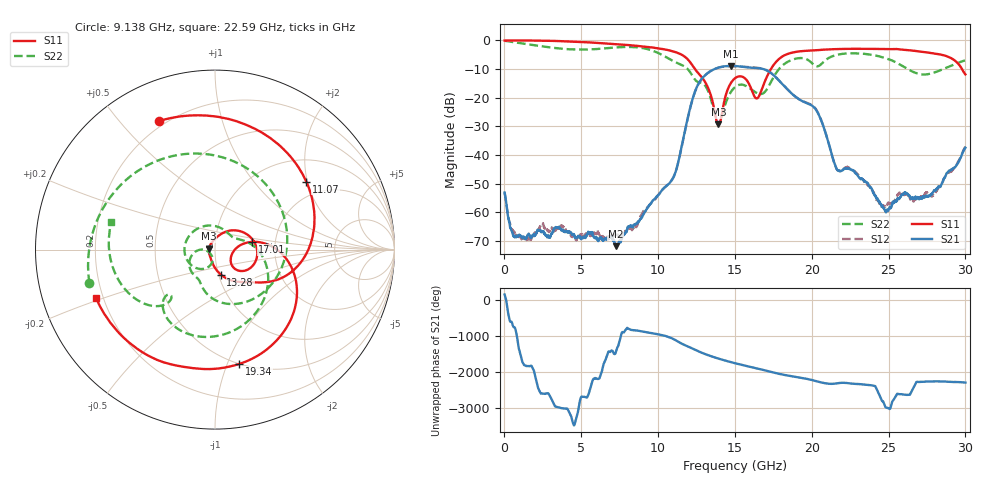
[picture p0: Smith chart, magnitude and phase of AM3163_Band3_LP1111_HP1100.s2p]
!Agilent Technologies,E8364B,MY43040894,A.07.50.67
!Agilent E8364B: A.07.50.67
!Date: Thursday, August 20, 2020 12:17:28
!Correction: S11(Full 2 Port(1,2))
!S21(Full 2 Port(1,2))
!S12(Full 2 Port(1,2))
!S22(Full 2 Port(1,2))
!S2P File: Measurements: S11, S21, S12, S22:
# Hz S  dB  R 50
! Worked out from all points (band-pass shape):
!   3201 points, 10 MHz to 30 GHz, reference 50 ohm
!   highest |S21| = -8.87 dB at 14.75 GHz (marker M1); lowest = -71.7 dB at 7.245 GHz (marker M2)
!   |S21| within 3 dB of the highest: 13.12 GHz to 17.47 GHz (4.35 GHz wide, 28.4 % of centre)
!   lowest |S11| = -29.3 dB at 13.93 GHz (marker M3), VSWR 1.07, Z = 46.7 + j0.464 ohm
!   |S11| at or under -10 dB: 12.41 GHz to 17.34 GHz (4.934 GHz wide, 33.2 % of centre); 29.78 GHz to end of sweep
!   |S22| runs from -29.2 to -0.1 dB; largest |S21 - S12| = 0.01
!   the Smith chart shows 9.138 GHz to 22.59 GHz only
!   S11 on the Smith chart (normalised r, x): 9.138 GHz: 0.17, +0.64; 11.07 GHz: 1.55, +1.97; 13.28 GHz: 1.03, -0.29; 17.01 GHz: 1.52, +0.14; 19.34 GHz: 0.50, -1.11; 22.59 GHz: 0.17, -0.19
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1e7  -0.05 -1.8  -53.03 149.4  -52.91 -149.2  -0.12 -5.1
1.247088e9  -0.00 -33.4  -68.45 20.4  -68.75 16.7  -1.12 -82.1
2.662241e9  -0.10 -71.2  -67.71 -81.2  -65.69 -149.1  -2.21 -162.3
5.014581e9  -0.54 -131.9  -68.96 -156.8  -67.96 123.3  -3.20 74.3
7.245088e9  -1.26 169.9  -71.75 -11.1  -67.82 34.8  -2.43 -49.6
8.182275e9  -1.66 143.3  -64.67 -96.7  -65.60 -145.1  -2.25 -104.2
9.138206e9  -2.15 113.5  -59.76 -166.8  -59.02 -169.4  -2.80 -165.0
1.000979e10  -2.75 82.4  -53.93 127.4  -53.86 127.2  -4.38 129.5
1.106881e10  -3.96 36.7  -46.83 -18.8  -46.91 -18.6  -7.41 25.9
1.186542e10  -6.25 -7.7  -28.56 165.4  -28.75 165.7  -9.67 -66.3
1.328058e10  -16.89 -76.8  -11.18 -93.2  -11.14 -92.3  -17.98 -168.6
1.392723e10  -29.27 171.7  -9.47 176.3  -9.47 176.4  -29.24 -138.7
1.475196e10  -14.72 32.0  -8.87 76.5  -9.00 77.2  -17.86 -122.5
1.5005e10  -13.18 13.3  -8.91 48.5  -9.02 49.7  -16.29 -141.6
1.701058e10  -13.48 11.7  -10.29 -157.0  -10.26 -156.7  -17.56 27.8
1.934418e10  -3.73 -77.9  -21.05 1.0  -20.99 1.9  -6.15 -108.1
2.000958e10  -3.49 -96.9  -22.71 -56.5  -22.53 -56.0  -7.89 -135.6
2.163092e10  -3.01 -136.2  -44.92 -149.5  -44.92 -154.8  -5.03 -161.1
2.258685e10  -2.92 -157.8  -45.03 -156.7  -45.03 -154.4  -4.48 165.1
2.500479e10  -3.02 145.3  -58.98 -119.1  -56.78 -3.4  -6.56 68.1
2.740399e10  -4.12 77.9  -54.27 -101.9  -53.27 -2.0  -11.87 -88.2
3e10  -11.83 -27.3  -37.41 -128.2  -37.02 -126.0  -6.96 131.0
